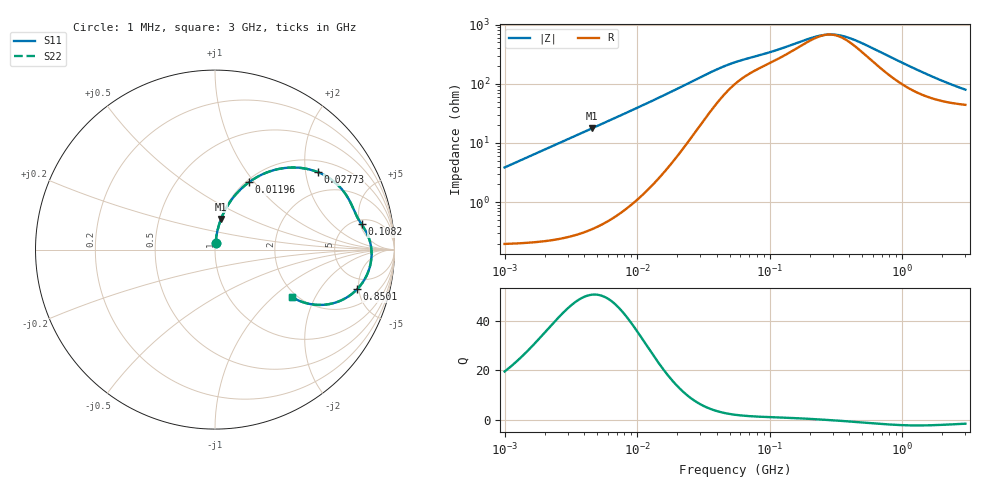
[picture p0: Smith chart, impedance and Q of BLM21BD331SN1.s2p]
! BLM21BD331SN1
# Hz S RI R 50
!Freq.(Hz) S11(Real) S11(Imag) S21(Real) S21(Imag) S12(Real) S12(Imag) S22(Real) S22(Imag)
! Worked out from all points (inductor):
!   401 points, 1 MHz to 3 GHz, reference 50 ohm
!   read as one part in series: L = 613 nH near 1.041 MHz
!   highest Q = 50.5 at 4.578 MHz (marker M1), where L = 615 nH
!   self-resonance near 275.6 MHz
!   S11 on the Smith chart (normalised r, x): 1 MHz: 1.00, +0.08; 11.96 MHz: 1.03, +0.94; 27.73 MHz: 1.31, +2.34; 108.2 MHz: 5.87, +5.28; 850.1 MHz: 3.52, -4.79; 3 GHz: 1.88, -1.33
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1000000  0.00344 0.0383  0.9966 -0.0383  0.9966 -0.0383  0.00344 0.0383
2097170  0.00867 0.08  0.9913 -0.08  0.9913 -0.08  0.00867 0.08
3823119  0.0242 0.1437  0.9758 -0.1437  0.9758 -0.1437  0.0242 0.1437
4577760  0.0336 0.1705  0.9664 -0.1705  0.9664 -0.1705  0.0336 0.1705
7858845  0.091 0.2762  0.909 -0.2762  0.909 -0.2762  0.091 0.2762
1.196486e7  0.1905 0.3761  0.8095 -0.3761  0.8095 -0.3761  0.1905 0.3761
1.461624e7  0.2629 0.4188  0.7371 -0.4188  0.7371 -0.4188  0.2629 0.4188
2.054061e7  0.4214 0.4572  0.5786 -0.4572  0.5786 -0.4572  0.4214 0.4572
2.773354e7  0.5718 0.432  0.4282 -0.432  0.4282 -0.432  0.5718 0.432
3.820236e7  0.6939 0.3505  0.3061 -0.3505  0.3061 -0.3505  0.6939 0.3505
5.477226e7  0.7605 0.2507  0.2395 -0.2507  0.2395 -0.2507  0.7605 0.2507
1.081723e8  0.817 0.1406  0.183 -0.1406  0.183 -0.1406  0.817 0.1406
2.094008e8  0.8633 0.0453  0.1367 -0.0453  0.1367 -0.0453  0.8633 0.0453
2.771263e8  0.8715 -0.000925  0.1285 0.000925  0.1285 0.000925  0.8715 -0.000925
3.523638e8  0.8717 -0.0432  0.1283 0.0432  0.1283 0.0432  0.8717 -0.0432
4.570858e8  0.8637 -0.0923  0.1363 0.0923  0.1363 0.0923  0.8637 -0.0923
8.005644e8  0.803 -0.2086  0.197 0.2086  0.197 0.2086  0.803 -0.2086
8.501091e8  0.7917 -0.221  0.2083 0.221  0.2083 0.221  0.7917 -0.221
1.218836e9  0.7016 -0.2837  0.2984 0.2837  0.2984 0.2837  0.7016 -0.2837
1.613037e9  0.6118 -0.307  0.3882 0.307  0.3882 0.307  0.6118 -0.307
2.134733e9  0.5201 -0.3013  0.4799 0.3013  0.4799 0.3013  0.5201 -0.3013
3e9  0.427 -0.2635  0.573 0.2635  0.573 0.2635  0.427 -0.2635
